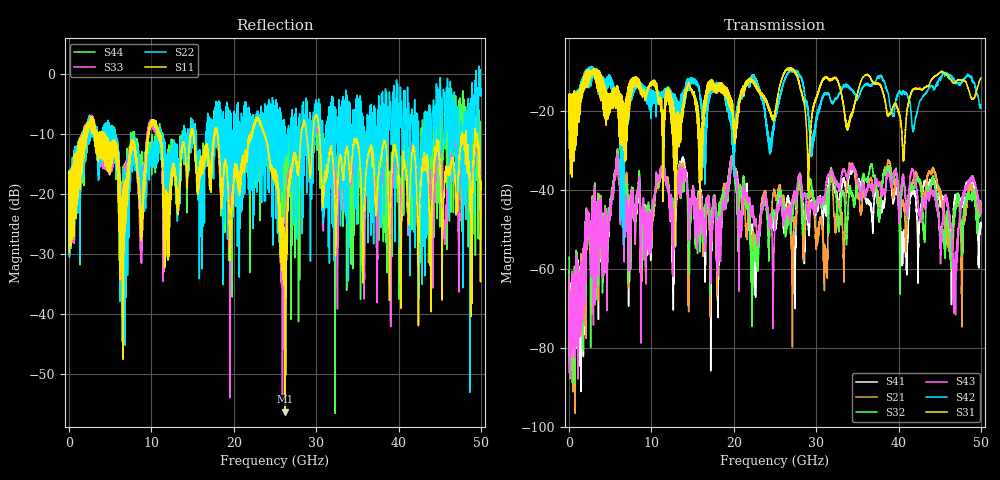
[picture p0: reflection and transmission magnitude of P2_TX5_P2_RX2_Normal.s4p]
!Keysight Technologies,N5225B,MY57041031,A.13.20.10
!Date: Friday, May 31, 2019 11:29:26
!Correction: S11(Full 4 Port(1,2,3,4))
!S12(Full 4 Port(1,2,3,4))
!S13(Full 4 Port(1,2,3,4))
!S14(Full 4 Port(1,2,3,4))
!S21(Full 4 Port(1,2,3,4))
!S22(Full 4 Port(1,2,3,4))
!S23(Full 4 Port(1,2,3,4))
!S24(Full 4 Port(1,2,3,4))
!S31(Full 4 Port(1,2,3,4))
!S32(Full 4 Port(1,2,3,4))
!S33(Full 4 Port(1,2,3,4))
!S34(Full 4 Port(1,2,3,4))
!S41(Full 4 Port(1,2,3,4))
!S42(Full 4 Port(1,2,3,4))
!S43(Full 4 Port(1,2,3,4))
!S44(Full 4 Port(1,2,3,4))
!S4P File: Measurements: <S11,S12,S13,S14>,
!<S21,S22,S23,S24>,
!<S31,S32,S33,S34>,
!<S41,S42,S43,S44>:
# Hz S  dB  R 50.0
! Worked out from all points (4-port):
!   5000 points, 10 MHz to 50 GHz, reference 50 ohm
!   strongest paths, dB at 10 MHz, 12.51 GHz, 25.01 GHz, 37.51 GHz, 50 GHz:
!     S31: -19.4, -17.8, -20.9, -13.2, -11.7
!     S42: -19.4, -15.8, -21.4, -11.2, -18.4
!     S43: -62.2, -46.7, -48.5, -39.0, -46.1
!     S32: -57.0, -44.1, -47.6, -43.3, -43.7
!     S21: -60.4, -44.6, -40.8, -41.6, -44.6
!     S41: -62.5, -49.3, -47.7, -43.0, -49.1
!   lowest |S11| = -56.2 dB at 26.24 GHz (marker M1), VSWR 1.00, Z = 50 + j0.155 ohm
!   |S11| at or under -10 dB: 4.42 GHz to 9.568 GHz (5.148 GHz wide, 73.6 % of centre); 23.74 GHz to 28.18 GHz (4.44 GHz wide, 17.1 % of centre); 30.41 GHz to 47.7 GHz (17.29 GHz wide, 44.3 % of centre)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
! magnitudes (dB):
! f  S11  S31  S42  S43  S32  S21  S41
! 10 MHz  -19.9  -19.4  -19.4  -62.2  -57.0  -60.4  -62.5
! 5.87 GHz  -13.7  -14.2  -17.9  -32.0  -31.2  -30.9  -31.7
! 19.83 GHz  -19.8  -19.3  -25.5  -32.6  -32.1  -31.7  -32.7
! 22.93 GHz  -7.1  -14.9  -13.9  -53.3  -57.8  -50.7  -57.2
! 26.24 GHz  -56.2  -9.9  -11.9  -46.2  -48.8  -45.4  -47.3
! 30.01 GHz  -6.8  -16.7  -23.1  -43.9  -44.0  -54.4  -44.2
! 50 GHz  -19.2  -11.7  -18.4  -46.1  -43.7  -44.6  -49.1
